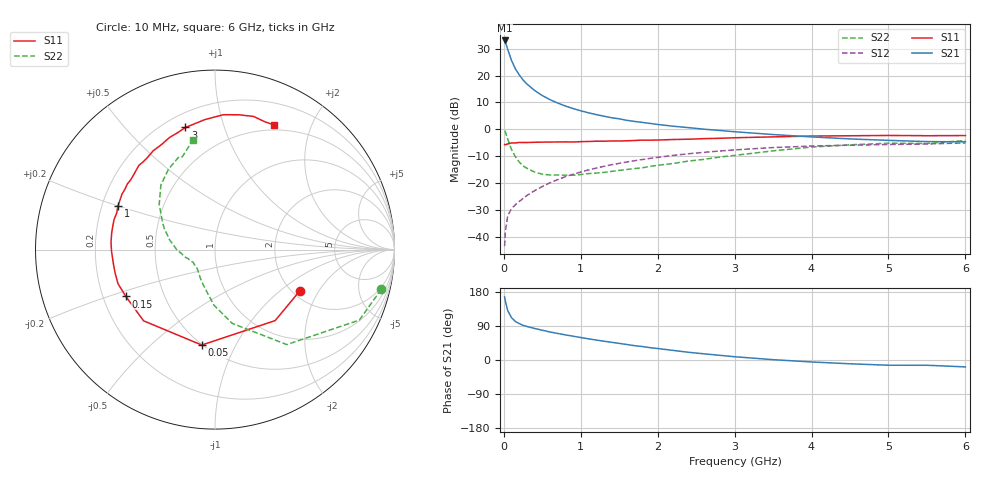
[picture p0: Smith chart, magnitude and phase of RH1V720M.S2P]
! SIEMENS Small Signal Semiconductors
! BFR106
! Si NPN RF Bipolar Junction Transistor in SOT23
! VCE = 1.75 V  IC = 20 mA
! Common Emitter S-Parameters:  August  1996
# GHz  S  MA  R  50
!  f  S11  S21  S12  S22
! GHz  MAG  ANG  MAG  ANG  MAG  ANG  MAG  ANG
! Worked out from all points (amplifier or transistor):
!   36 points, 10 MHz to 6 GHz, reference 50 ohm
!   highest |S21| = 33.0 dB at 10 MHz (marker M1)
!   |S21| within 3 dB of that: start of sweep to 46.72 MHz
!   unconditionally stable (mu >= 1): 354.7 MHz to 2.565 GHz; 4.839 GHz to end of sweep
!   at 250 MHz: K = 0.91, MSG = 22.0 dB, |S12| = -25.6 dB
!   at 1.4 GHz: K = 1.08, MAG = 7.0 dB, |S12| = -13.1 dB
!   at 6 GHz: K = 1.02, MAG = -0.6 dB, |S12| = -5.0 dB
!   S11 on the Smith chart (normalised r, x): 10 MHz: 2.17, -1.39; 50 MHz: 0.50, -0.74; 150 MHz: 0.30, -0.23; 1 GHz: 0.27, +0.20; 3 GHz: 0.28, +0.75; 6 GHz: 0.44, +1.49
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0.01  0.525 -26.2  44.81 166.5  0.0068 81.1  0.9525 -13.4
0.02  0.5185 -49.7  41.87 155.4  0.0129 71.4  0.8952 -26.0
0.05  0.537 -97.9  30.66 130.7  0.0247 55.8  0.6635 -52.9
0.1  0.562 -135.1  19.05 111.5  0.0341 50.2  0.4225 -76.8
0.15  0.5611 -152.3  13.35 101.7  0.04 51.1  0.3107 -91.0
0.2  0.5728 -160.7  10.29 96.0  0.046 54.0  0.2482 -99.3
0.25  0.5715 -167.2  8.276 91.5  0.0522 56.0  0.2098 -107.7
0.3  0.5717 -172.0  6.949 88.5  0.0596 58.6  0.1899 -113.7
0.4  0.5768 -179.3  5.284 83.2  0.073 61.4  0.1615 -123.9
0.5  0.5807 175.9  4.246 78.5  0.0871 63.1  0.1473 -131.3
0.6  0.5832 170.8  3.566 74.0  0.1023 63.5  0.1425 -136.4
0.7  0.5845 166.6  3.087 70.0  0.1168 63.8  0.1423 -141.7
0.8  0.5868 163.4  2.719 66.3  0.1325 63.3  0.1414 -146.5
1  0.5929 155.7  2.216 59.3  0.1619 61.9  0.1455 -152.6
1.1  0.5971 152.4  2.035 55.9  0.177 61.0  0.1512 -155.8
1.6  0.6146 137.8  1.473 40.8  0.2486 54.5  0.1806 -170.0
2.2  0.6493 122.0  1.147 25.3  0.3289 45.6  0.233 173.8
3  0.7 103.6  0.905 8.6  0.4169 32.7  0.3292 152.6
3.5  0.7267 94.4  0.803 0.9  0.4604 24.9  0.4 141.0
4.5  0.7627 80.0  0.666 -10.0  0.5099 10.0  0.5177 120.0
5.5  0.7645 68.7  0.594 -13.9  0.5364 1.0  0.5483 109.4
6  0.7684 64.6  0.589 -18.2  0.5622 -6.0  0.6225 101.4
